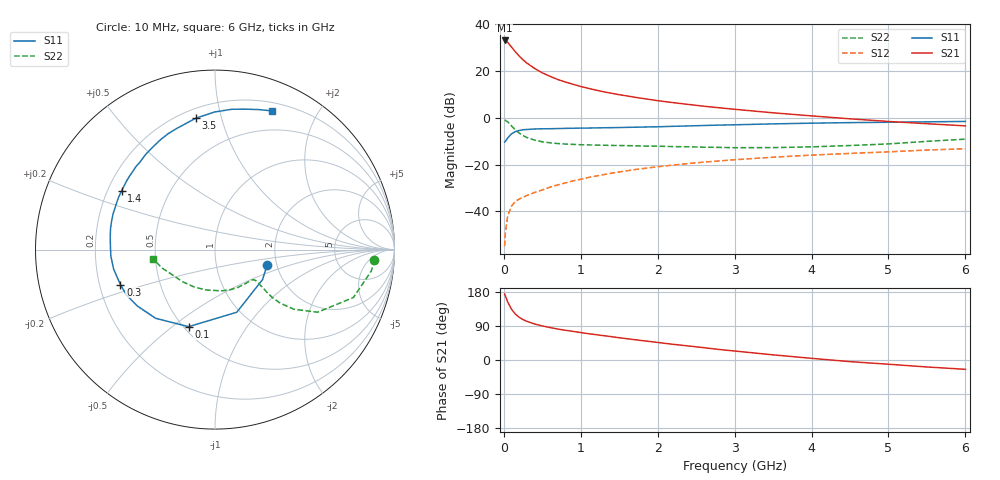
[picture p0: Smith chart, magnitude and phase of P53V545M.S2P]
! SIEMENS Small Signal Semiconductors
! BFP183
! Si NPN RF Bipolar Junction Transistor in SOT143
! VCE = 3.5 V  IC = 45 mA
! Common Emitter S-Parameters:  March  1996
# GHz  S  MA  R  50
!  f  S11  S21  S12  S22
! GHz  MAG  ANG  MAG  ANG  MAG  ANG  MAG  ANG
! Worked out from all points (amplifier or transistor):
!   36 points, 10 MHz to 6 GHz, reference 50 ohm
!   highest |S21| = 33.0 dB at 10 MHz (marker M1)
!   |S21| within 3 dB of that: start of sweep to 103.9 MHz
!   unconditionally stable (mu >= 1): start of sweep to 12.57 MHz; 408.7 MHz to end of sweep
!   at 250 MHz: K = 0.78, MSG = 29.4 dB, |S12| = -34.0 dB
!   at 1.4 GHz: K = 1.29, MAG = 13.8 dB, |S12| = -23.7 dB
!   at 6 GHz: K = 1.02, MAG = 4.0 dB, |S12| = -13.2 dB
!   S11 on the Smith chart (normalised r, x): 10 MHz: 1.78, -0.33; 100 MHz: 0.53, -0.57; 300 MHz: 0.29, -0.16; 1.4 GHz: 0.26, +0.27; 3.5 GHz: 0.26, +0.83; 6 GHz: 0.28, +1.45
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0.01  0.3027 -16.2  44.92 174.3  0.0018 73.2  0.8901 -3.6
0.02  0.3132 -32.1  44.57 168.9  0.0035 77.3  0.8792 -7.8
0.05  0.3695 -70.8  41 153.1  0.008 74.4  0.816 -19.1
0.1  0.4539 -108.9  32.38 133.9  0.013 57.8  0.6696 -31.4
0.15  0.5058 -130.8  25.68 121.1  0.0163 53.1  0.5508 -37.1
0.2  0.5345 -143.9  20.81 112.7  0.0183 52.2  0.4702 -39.4
0.25  0.5543 -152.8  17.27 106.5  0.0199 51.8  0.4163 -39.9
0.3  0.562 -159.7  14.73 102.0  0.0219 51.7  0.3781 -39.5
0.4  0.5752 -169.2  11.33 95.0  0.0253 54.7  0.3328 -38.4
0.5  0.5813 -176.4  9.128 89.9  0.0286 55.8  0.3066 -37.7
0.6  0.583 178.1  7.707 85.6  0.0329 57.7  0.2915 -37.3
0.7  0.588 173.1  6.577 81.8  0.0367 59.1  0.2812 -37.4
0.8  0.5935 168.8  5.812 78.4  0.0405 59.4  0.2744 -37.8
1.1  0.6033 157.6  4.251 69.4  0.053 60.1  0.2623 -41.1
1.4  0.6147 147.9  3.339 61.6  0.0653 59.3  0.2562 -45.9
1.7  0.6285 139.0  2.746 53.6  0.078 57.4  0.2521 -52.0
2.2  0.6564 126.0  2.106 41.4  0.0974 53.1  0.2419 -63.4
2.8  0.6968 111.9  1.634 27.7  0.1195 47.2  0.2328 -80.1
3.5  0.7399 98.3  1.276 13.6  0.1434 40.7  0.2302 -102.5
4.5  0.7874 83.2  0.949 -4.3  0.1729 30.9  0.2551 -135.9
5.5  0.8182 72.4  0.746 -18.4  0.2044 22.5  0.3135 -161.1
6  0.8348 67.8  0.671 -24.6  0.2176 17.6  0.3491 -171.7
